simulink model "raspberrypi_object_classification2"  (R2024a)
settings: Solver=ode45  StartTime=0.0  StopTime=10.0  RelTol=1e-3  EnableMultiTasking=on
model workspace (MAT data in the model file):
  RGBData = [62 63 65 64 60 62 65 62 60 59 59 59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]
libraries: raspberrypiAVlib x2, deeplib x1, visiontextngfix x1

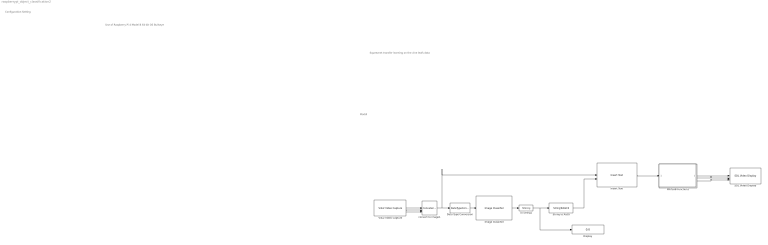
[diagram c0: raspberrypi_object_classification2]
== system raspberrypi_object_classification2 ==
  note: Squeeznet transfer learning on the vine leafs data
  note: Use of Raspberry Pi 4 Model B 64-bit OS Bullseye
  note: Moddl
  note: Configuration Setting
  Data Type Conversion : DataTypeConversion  OutDataTypeStr=single
  Display : Display
  Image Classifier : deeplib/Image Classifier  Network=Network from MAT-file  NetworkFunction=resnet50  NetworkFilePath=C:\work\PASS\Tonnerre\SI-IA-VigneNette-main\SI-IA-VigneNette-main\2-TransferLearning\monSqueeze.mat  NetworkClassesVariable=classNames  MiniBatchSize=128  ResizeInput=on  Classification=on  Predictions=off  ForceInterpretedSim=off  PredictMode=All probabilities and labels  K=5
  Insert Text : visiontextngfix/Insert Text  inputType=Obsolete  theText='%s'  getTextLocFrom=Specify via dialog  textLoc=[1 1]  getTextColorFrom=Specify via dialog  textColor=[255,255,0]  getTextIntensityFrom=Specify via dialog  textIntensity=0  getTextOpacityFrom=Specify via dialog  textOpacity=1.0  dummyVar2=0  dummyVar3=0  dummyVar4=0  imagePorts=One multidimensional signal  isInputTransposed=on  fontFace=LucidaSansRegular  dummyVar1=0  blockFontSize=18  antiAliased=off
  MATLAB Function1 : MATLAB Function  TreatAsAtomicUnit=on
  SDL Video Display : raspberrypiAVlib/SDL Video Display  title=SDL Video Display  pixelFormat=RGB  pixelOrder=Planar  rowMajor=on  blockPlatform=Raspberry Pi
  String to ASCII : StringToASCII
  To String1 : ToString
  V4L2 Video Capture : raspberrypiAVlib/V4L2 Video Capture  DeviceName=/dev/video0  Resolution=320x240  CustomResolution=[ 320, 240 ]  PixelFormat=RGB  SampleTime=0.1  pixelOrder=planar  simOutput=Colorbars  imSizeSelection=320x240  imSize=[640, 480]  roi=[0, 0, 640, 480]  m_devName='/dev/video0'  blockPlatform=LINUX  HorizontalFlip=off  VerticalFlip=off  Brightness=0.5  Saturation=0.5  Contrast=0.5  Sharpness=0.5  CameraPan=0  CameraTilt=0  CameraZoom=0.5  EnableManualFocus=on  ManualFocus=0.5
  convert to image1 : Concatenate  NumInputs=3  Mode=Multidimensional array  ConcatenateDimension=3
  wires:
  V4L2 Video Capture/3 -> convert to image1/3
  V4L2 Video Capture/2 -> convert to image1/2
  V4L2 Video Capture/1 -> convert to image1/1
  convert to image1/1 -> Insert Text/1, Data Type Conversion/1
  Data Type Conversion/1 -> Image Classifier/1
  To String1/1 -> Display/1, String to ASCII/1
  MATLAB Function1/3(b) -> SDL Video Display/3
  String to ASCII/1 -> Insert Text/2
  MATLAB Function1/1(r) -> SDL Video Display/1
  Image Classifier/1 -> To String1/1
  MATLAB Function1/2(g) -> SDL Video Display/2
  Insert Text/1 -> MATLAB Function1/1(i)

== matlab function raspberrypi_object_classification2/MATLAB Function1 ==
function [r,g,b] = ImageToRGB(i)
%#codegen
r =i(:,:,1);
g =i(:,:,2);
b =i(:,:,3);
end
